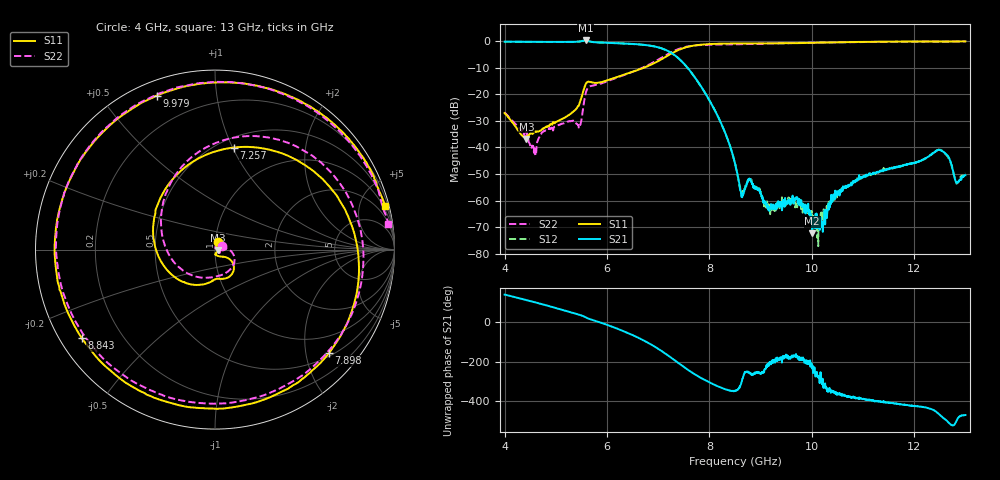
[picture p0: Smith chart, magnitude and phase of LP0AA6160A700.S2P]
! FILE NAME
! DATE 09/10/2014  14:44
! CORRECTED  DATA
# GHz  S  MA  R  50.00
!  FREQ  S11M  S11A  S21M  S21A  S12M  S12A  S22M  S22A
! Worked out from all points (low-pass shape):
!   1601 points, 4 GHz to 13 GHz, reference 50 ohm
!   highest |S21| = 0.13 dB at 5.586 GHz (marker M1); lowest = -72.1 dB at 10.01 GHz (marker M2)
!   |S21| within 3 dB of the highest: start of sweep to 7.075 GHz
!   lowest |S11| = -36.8 dB at 4.428 GHz (marker M3), VSWR 1.03, Z = 51.4 - j0.322 ohm
!   |S11| at or under -10 dB: start of sweep to 6.732 GHz
!   |S22| runs from -43.1 to -0.2 dB; largest |S21 - S12| = 0.007
!   S11 on the Smith chart (normalised r, x): 4 GHz: 1.03, +0.08; 7.257 GHz: 0.59, +1.01; 7.898 GHz: 0.57, -2.48; 8.843 GHz: 0.06, -0.30; 9.979 GHz: 0.06, +0.69; 13 GHz: 0.73, +7.82
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4  0.0443 67.0  0.9643 136.9  0.9649 137.0  0.04514 30.4
4.4275  0.0144 -12.6  0.9591 108.9  0.9608 108.9  0.0197 41.2
4.585  0.01955 -68.3  0.9561 98.4  0.9552 98.1  0.009297 61.3
5.501875  0.08729 -33.2  0.9859 31.6  0.9893 31.6  0.03329 0.2
5.58625  0.1556 -48.2  1.015 22.0  1.015 21.6  0.1061 -14.8
6.48625  0.2613 -138.9  0.8767 -65.4  0.876 -65.3  0.2593 -174.3
7.00375  0.4195 136.3  0.7539 -136.5  0.7557 -136.6  0.4469 123.3
7.256875  0.578 79.6  0.5945 178.4  0.5942 178.4  0.6134 85.0
7.583125  0.7745 9.6  0.3042 117.6  0.3039 117.7  0.7871 28.2
7.898125  0.8575 -42.2  0.1121 68.6  0.1123 68.5  0.8414 -23.8
8.5  0.8923 -112.3  0.004949 13.5  0.004991 10.2  0.8611 -110.2
8.635  0.8923 -126.0  0.001388 60.0  0.001444 61.3  0.8664 -127.7
8.843125  0.8914 -146.5  0.002022 93.1  0.002082 97.7  0.8745 -152.9
9.338125  0.895 165.2  0.0009422 176.4  0.000755 173.7  0.8982 156.2
9.709375  0.9055 131.9  0.001175 -173.6  0.0007667 -173.0  0.9142 126.2
9.979375  0.9172 110.8  0.0003825 152.4  0.0004779 137.7  0.9241 108.2
10.00188  0.9186 109.2  0.0004639 141.0  0.0004716 141.6  0.9244 106.9
10.0075  0.9194 108.7  0.0002472 133.1  0.0005352 129.5  0.9242 106.6
11.50375  0.9662 43.1  0.003878 -45.7  0.003951 -44.8  0.9576 42.0
12.49375  0.9714 22.0  0.008983 -106.7  0.009045 -106.7  0.9647 16.6
12.83125  0.9756 16.8  0.002169 -136.6  0.002095 -134.5  0.9723 10.9
13  0.9769 14.4  0.003014 -108.9  0.003299 -109.1  0.9758 8.3
